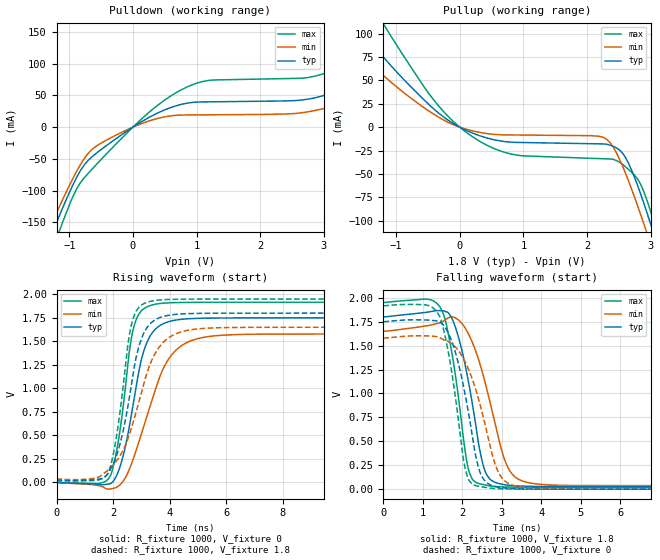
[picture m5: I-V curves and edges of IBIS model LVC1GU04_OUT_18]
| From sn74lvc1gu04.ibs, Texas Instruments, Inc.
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[Model]   LVC1GU04_OUT_18
Model_type  Output
Vref =   0
Rref =   1000
Cref =   30p
Vmeas =   0.9
| variable   typ   min   max
C_comp   8.24pF   4.14pF   13.04pF
| C_pullup   8.04pF   5.33pF   10.37pF
| C_pulldown   8.44pF   4.14pF   13.04pF
[Temperature Range]   40   100   -40
| Ambient temperature   25   85   -40
[Voltage range]   1.8   1.65   1.95
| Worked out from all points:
|   slope of the pulldown table from 0 to 0.27 V, typ, clamps not added: 16.6 ohm
|   slope of the pullup table from 0 to 0.27 V, typ, clamps not added: 33.1 ohm
|   rising waveform, R_fixture 1000, V_fixture 0: 20-80 % time 679ps typ, 1.08ns min, 494ps max; typ from 0 V to 1.75 V
|   falling waveform, R_fixture 1000, V_fixture 1.8: 20-80 % time 464ps typ, 598ps min, 396ps max; typ from 1.8 V to 0.027 V
|   rising waveform, R_fixture 1000, V_fixture 1.8: 20-80 % time 694ps typ, 1.03ns min, 501ps max; typ from 0.027 V to 1.8 V
|   falling waveform, R_fixture 1000, V_fixture 0: 20-80 % time 494ps typ, 643ps min, 406ps max; typ from 1.75 V to 0 V
[Pulldown]
| LVC1GU04_OUT_18
|   Voltage   I(typ)   I(min)   I(max)
-5.5V     -1.241A    -1.151A    -1.389A
-1.385V   -195.8mA   -176.6mA   -228mA
-1.175V   -144.3mA   -129.6mA   -169.3mA
-845mV    -72.21mA   -62.67mA   -90.77mA
-590mV    -42.45mA   -30.94mA   -60.69mA
735mV     35.27mA    19.06mA    57.56mA
1.195V    39.91mA    19.44mA    73.76mA
2.885V    46.82mA    26.69mA    80.97mA
4.235V    111.4mA    81.74mA    163.2mA
4.82V     154.7mA    117.8mA    220.3mA
5.44V     207.6mA    162mA      290.4mA
11V       864.7mA    712.8mA    1.162A
[Pullup]
| LVC1GU04_OUT_18
|   Voltage   I(typ)   I(min)   I(max)
-5.5V     528.9mA    421.5mA    733.8mA
-1.985V   141.7mA    107.2mA    204.6mA
-1.575V   105.5mA    78.75mA    153.7mA
-1.2V     74.83mA    55.07mA    110.3mA
-335mV    15.2mA     10.75mA    22.9mA
285mV     -8.519mA   -5.256mA   -13.94mA
890mV     -16.32mA   -8.395mA   -29.83mA
2.285V    -18.08mA   -11.93mA   -33.84mA
2.605V    -32.54mA   -49.2mA    -42.36mA
2.92V     -86.82mA   -108.8mA   -73.89mA
3.095V    -123.9mA   -145mA     -110.9mA
11V       -2.109A    -2.018A    -2.277A
[Ramp]
| LVC1GU04_OUT_18
| variable   typ   min   max
dV/dt_r   1.06/6.93E-10   0.99/1.12E-09   1.16/5.01E-10
dV/dt_f   1.10/4.95E-10   1.06/6.78E-10   1.18/4.12E-10
R_load = 1000
[Rising Waveform]
| LVC1GU04_OUT_18
R_fixture =   1000
C_fixture =   0
L_fixture =   0
V_fixture =   0
V_fixture_min = 0
V_fixture_max = 0
|   Time   V(typ)   V(min)   V(max)
0s        32.52pV    7.411nV    2.092nV
1.89ns    -15.18mV   -71.79mV   62.18mV
2.305ns   225.2mV    -7.625mV   684.8mV
2.585ns   611.8mV    145.3mV    1.412V
2.74ns    881.3mV    272.5mV    1.66V
3.115ns   1.424V     624.3mV    1.853V
3.625ns   1.662V     1.101V     1.901V
4.505ns   1.737V     1.47V      1.914V
6.275ns   1.749V     1.571V     1.915V
50ns      1.749V     1.578V     1.915V
[Falling Waveform]
| LVC1GU04_OUT_18
R_fixture =   1000
C_fixture =   0
L_fixture =   0
V_fixture =   1.8
V_fixture_min = 1.65
V_fixture_max = 1.95
|   Time   V(typ)   V(min)   V(max)
0s        1.8V       1.65V      1.95V
1.285ns   1.861V     1.723V     1.962V
1.525ns   1.862V     1.757V     1.824V
1.69ns    1.817V     1.798V     1.528V
2.17ns    1.089V     1.61V      185.3mV
2.515ns   269.7mV    1.21V      49.98mV
2.81ns    74.1mV     720.3mV    28.95mV
3.285ns   36.78mV    147.3mV    21.21mV
4.305ns   27.41mV    42.58mV    19.77mV
50ns      26.95mV    37.1mV     19.71mV
[Rising Waveform]
| LVC1GU04_OUT_18
R_fixture =   1000
C_fixture =   0
L_fixture =   0
V_fixture =   1.8
V_fixture_min = 1.65
V_fixture_max = 1.95
|   Time   V(typ)   V(min)   V(max)
0s        26.95mV    37.1mV     19.71mV
1.82ns    95.03mV    127.6mV    97.04mV
2.26ns    427mV      289.8mV    782.5mV
2.525ns   811.9mV    465.4mV    1.466V
2.685ns   1.106V     614.9mV    1.718V
3.02ns    1.542V     973.2mV    1.889V
3.515ns   1.734V     1.385V     1.936V
4.315ns   1.79V      1.592V     1.948V
5.97ns    1.8V       1.647V     1.95V
50ns      1.8V       1.65V      1.95V
[Falling Waveform]
| LVC1GU04_OUT_18
R_fixture =   1000
C_fixture =   0
L_fixture =   0
V_fixture =   0
V_fixture_min = 0
V_fixture_max = 0
|   Time   V(typ)   V(min)   V(max)
0s        1.749V     1.578V     1.915V
1.195ns   1.764V     1.6V       1.909V
1.56ns    1.693V     1.554V     1.604V
1.825ns   1.428V     1.484V     959.7mV
2.105ns   912.6mV    1.3V       163.5mV
2.42ns    211.6mV    927.7mV    29.57mV
2.745ns   38.9mV     380.2mV    9.296mV
3.13ns    10.23mV    68.82mV    1.959mV
4.21ns    371.7uV    3.02mV     52.94uV
50ns      4.444nV    12.61nV    8.059nV
